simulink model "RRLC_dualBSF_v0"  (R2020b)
settings: Solver=VariableStepAuto  StartTime=0.0  StopTime=1  MaxStep=1e-4  RelTol=1e-5
libraries: fl_lib x10, nesl_utility x3

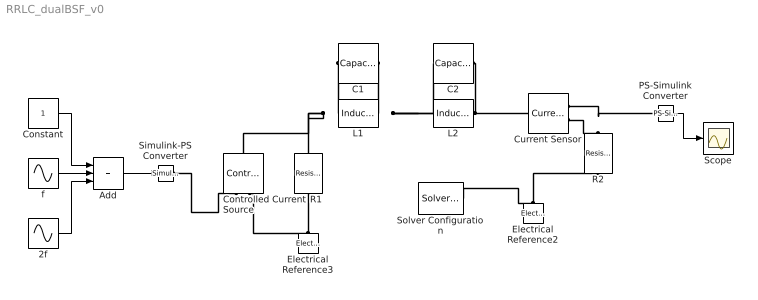
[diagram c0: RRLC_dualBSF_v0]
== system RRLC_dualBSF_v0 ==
  2f : Sin  Frequency=2e4  Phase=-pi/2  SampleTime=0
  Add : Sum  Inputs=+++
  C1 : fl_lib/Electrical/Electrical Elements/Capacitor  c=5e-6 F  r=0 Ohm  g=1e-6 1/Ohm  i_specify=off  i_priority=None  i=0 A  i_nominal_specify=off  i_nominal_unit=A  i_nominal_value=1  v_specify=off  v_priority=None  v=0 V  v_nominal_specify=off  v_nominal_unit=V  v_nominal_value=1  vc_specify=off  vc_priority=High  vc=0 V  vc_nominal_specify=off  vc_nominal_unit=V  vc_nominal_value=1
  C2 : fl_lib/Electrical/Electrical Elements/Capacitor  c=10e-6 F  r=0 Ohm  g=1e-6 1/Ohm  i_specify=off  i_priority=None  i=0 A  i_nominal_specify=off  i_nominal_unit=A  i_nominal_value=1  v_specify=off  v_priority=None  v=0 V  v_nominal_specify=off  v_nominal_unit=V  v_nominal_value=1  vc_specify=off  vc_priority=High  vc=0 V  vc_nominal_specify=off  vc_nominal_unit=V  vc_nominal_value=1
  Constant : Constant
  Controlled Current Source : fl_lib/Electrical/Electrical Sources/Controlled Current Source
  Current Sensor : fl_lib/Electrical/Electrical Sensors/Current Sensor
  Electrical Reference2 : fl_lib/Electrical/Electrical Elements/Electrical Reference
  Electrical Reference3 : fl_lib/Electrical/Electrical Elements/Electrical Reference
  L1 : fl_lib/Electrical/Electrical Elements/Inductor  l=0.5e-3 H  r=1e-6 Ohm  g=0 1/Ohm  i_specify=off  i_priority=None  i=0 A  i_nominal_specify=off  i_nominal_unit=A  i_nominal_value=1  v_specify=off  v_priority=None  v=0 V  v_nominal_specify=off  v_nominal_unit=V  v_nominal_value=1  i_L_specify=off  i_L_priority=High  i_L=0 A  i_L_nominal_specify=off  i_L_nominal_unit=A  i_L_nominal_value=1
  L2 : fl_lib/Electrical/Electrical Elements/Inductor  l=1e-3 H  r=1e-6 Ohm  g=0 1/Ohm  i_specify=off  i_priority=None  i=0 A  i_nominal_specify=off  i_nominal_unit=A  i_nominal_value=1  v_specify=off  v_priority=None  v=0 V  v_nominal_specify=off  v_nominal_unit=V  v_nominal_value=1  i_L_specify=off  i_L_priority=High  i_L=0 A  i_L_nominal_specify=off  i_L_nominal_unit=A  i_L_nominal_value=1
  PS-Simulink Converter : nesl_utility/PS-Simulink Converter  PhysicalDomain=network_engine_domain  SubClassName=ps_output  LeftPortType=input  RightPortType=output  PseudoPeriodic=off  Frequencies=[]  Unit=inherit  AffineConversion=off
  R1 : fl_lib/Electrical/Electrical Elements/Resistor  R=1 kOhm  i_specify=off  i_priority=None  i=0 A  i_nominal_specify=off  i_nominal_unit=A  i_nominal_value=1  v_specify=off  v_priority=None  v=0 V  v_nominal_specify=off  v_nominal_unit=V  v_nominal_value=1
  R2 : fl_lib/Electrical/Electrical Elements/Resistor  R=1 kOhm  i_specify=off  i_priority=None  i=0 A  i_nominal_specify=off  i_nominal_unit=A  i_nominal_value=1  v_specify=off  v_priority=None  v=0 V  v_nominal_specify=off  v_nominal_unit=V  v_nominal_value=1
  Scope : Scope
  Simulink-PS Converter : nesl_utility/Simulink-PS Converter  PhysicalDomain=network_engine_domain  SubClassName=ps_input  LeftPortType=input  RightPortType=output  PseudoPeriodic=off  Frequencies=[]  NoiseDistribution=none  NoiseParameters=[]  Unit=1  AffineConversion=off  FilteringAndDerivatives=provide  SimscapeFilterOrder=1  InputFilterTimeConstant=0.001  UdotUserProvided=0
  Solver Configuration : nesl_utility/Solver Configuration  PhysicalDomain=network_engine_domain  SubClassName=solver  LeftPortType=input  RightPortType=generic  Tones=[]  Harmonics=[]  SimulateNoise=off  Profile=off  UseLocalSampling=off  EnableSwitchedLinearOptims=on  FrequencyDomain=off  UseCCode=off  RelTol=0.001  AbsTol=1e-06  MinStep=1e-09  ToWorkspace=off  RevertToSquareIcSolve=off  NumHomotopyIterations=100  PhasorMode=off  PhasorModeNumHarmonics=1  DoDC=off  ResidualTolerance=1e-09  UseLocalSolver=off  LocalSolverChoice=NE_BACKWARD_EULER_ADVANCER  LocalSolverSampleTime=1e-5  DoFixedCost=off  MaxNonlinIter=3  MaxModeIter=2  ComputeImpulses=off  ImpulseIterations=2  LinearAlgebra=auto  EquationFormulation=NE_TIME_EF  DelaysMemoryBudget=1024  AutomaticFiltering=on  FilteringTimeConstant=0.001  PartitionStorageMethod=AS_NEEDED  PartitionMemoryBudget=1024  PartitionMethod=ROBUST
  f : Sin  Frequency=1e4  SampleTime=0
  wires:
  PS-Simulink Converter/1 -> Scope/1
  2f/1 -> Add/3
  Constant/1 -> Add/1
  f/1 -> Add/2
  Add/1 -> Simulink-PS Converter/1
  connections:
  Simulink-PS Converter/RConn1 -- Controlled Current Source/RConn1
  Electrical Reference3/LConn1 -- R1/RConn1 -- Controlled Current Source/RConn2
  Electrical Reference2/LConn1 -- Solver Configuration/RConn1 -- R2/RConn1
  L2/RConn1 -- Current Sensor/LConn1 -- C2/RConn1
  C1/LConn1 -- Controlled Current Source/LConn1 -- R1/LConn1 -- L1/LConn1
  C1/RConn1 -- C2/LConn1 -- L2/LConn1 -- L1/RConn1
  Current Sensor/RConn2 -- R2/LConn1
  Current Sensor/RConn1 -- PS-Simulink Converter/LConn1
